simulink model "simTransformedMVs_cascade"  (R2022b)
settings: Solver=ode15s  StartTime=0.0  StopTime=tsim  RelTol=1e-3
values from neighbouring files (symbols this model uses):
  Kparu1 = [0 1]    [runTransformedMVs.m]    (also in runTransformedMVsIS.m)
  Kparu2 = [1 0]    [runTransformedMVs.m]    (also in runTransformedMVsIS.m)
  Ku1 = 1/ku1*1/(tauCu1)    (= -0.05)    [runTransformedMVs.m]    (also in runTransformedMVsIS.m = -2)
  Ku2 = 1/ku2*1/(tauCu2)    (= 0.5)    [runTransformedMVs.m]    (also in runTransformedMVsIS.m = 1)
  p = [V;A(i);B(i)]    [runTransformedMVs.m]    (also in runTransformedMVsIS.m; Main.m = [N, Fc0, rhoc, rhoh,U,A,cpc,cph]; Main_OL.m = [N, Fc0, rhoc, rhoh,U,A,cpc,cph]; runTestCalcBlk.m = [N, Fc0, rhoc, rhoh,U,A,cpc,cph])
  q10 = 5    [runTransformedMVs.m]    (also in runTransformedMVsIS.m)
  q1f = q10*1    (= 5)    [runTransformedMVs.m]    (also in runTransformedMVsIS.m)
  q1max = 10    [runTransformedMVs.m]    (also in runTransformedMVsIS.m)
  q20 = 5    [runTransformedMVs.m]    (also in runTransformedMVsIS.m)
  q2f = q20*1    (= 5)    [runTransformedMVs.m]    (also in runTransformedMVsIS.m = 5.5)
  q2max = 10    [runTransformedMVs.m]    (also in runTransformedMVsIS.m)
  T0 = 35    [runTransformedMVs.m]    (also in runTransformedMVsIS.m; H2P_Turbine_driven.m = param(9); runTD.m = 318; H2P_Boiler_driven.m = param(9))
  T10 = 20    [runTransformedMVs.m]    (also in runTransformedMVsIS.m)
  T1f = T10-5    (= 15)    [runTransformedMVs.m]    (also in runTransformedMVsIS.m = 25)
  T1fm = T10    (= 20)    [runTransformedMVs.m]    (also in runTransformedMVsIS.m = 25)
  T20 = 50    [runTransformedMVs.m]    (also in runTransformedMVsIS.m)
  T2f = T20    (= 50)    [runTransformedMVs.m]    (also in runTransformedMVsIS.m = 70)
  T2fm = T20    (= 50)    [runTransformedMVs.m]    (also in runTransformedMVsIS.m = 70)
  tauTs = 0.1    [runTransformedMVs.m]    (also in runTransformedMVsIS.m)
  td1 = 100    [runTransformedMVs.m]    (also in runTransformedMVsIS.m = 200)
  td2 = 150    [runTransformedMVs.m]    (also in runTransformedMVsIS.m = 300)
  tv1 = 50    [runTransformedMVs.m]    (also in runTransformedMVsIS.m = 100)
  tv2 = 50    [runTransformedMVs.m]    (also in runTransformedMVsIS.m = 100)
  v10 = q0    (= 10)    [runTransformedMVs.m]    (also in runTransformedMVsIS.m)
  v1f = q0    (= 10)    [runTransformedMVs.m]    (also in runTransformedMVsIS.m = 15)
  v20 = B(i)^(-1)*(f20-A(i)*T0)    [runTransformedMVs.m]    (also in runTransformedMVsIS.m; runTransfOL.m = v00)
  v2f = v20    [runTransformedMVs.m]    (also in runTransformedMVsIS.m)
undefined symbols (not defined in the file or in its folder): InputTransfD, TempMixDAE

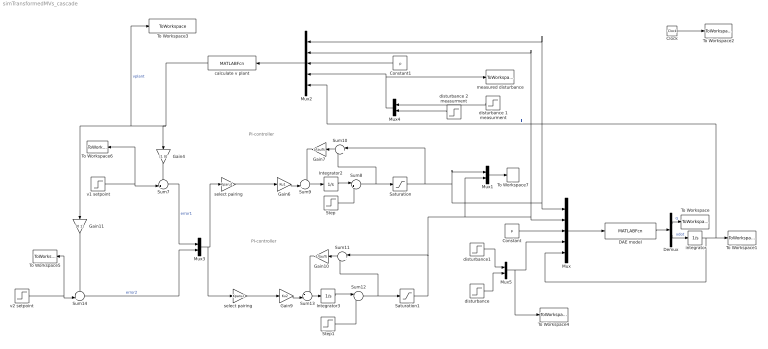
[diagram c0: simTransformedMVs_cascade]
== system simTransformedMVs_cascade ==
  note: PI-controller
  note: PI-controller
  " integrator" : Integrator  InitialCondition=T0
  Clock : Clock
  Constant : Constant  Value=p
  Constant1 : Constant  Value=p
  DAE model : MATLABFcn  MATLABFcn=TempMixDAE(u(1:2), u(3:5),u(6:7),u(8))  OutputDimensions=2
  Demux : Demux  Outputs=2
  Gain10 : Gain  Gain=1/tauTs  Multiplication=Matrix(K*u)
  Gain11 : Gain  Gain=[0 1]  Multiplication=Matrix(K*u)
  Gain4 : Gain  Gain=[1 0]  Multiplication=Matrix(K*u)
  Gain6 : Gain  Gain=Ku1  Multiplication=Matrix(K*u)
  Gain7 : Gain  Gain=1/tauTs  Multiplication=Matrix(K*u)
  Gain9 : Gain  Gain=Ku2  Multiplication=Matrix(K*u)
  Integrator2 : Integrator
  Integrator3 : Integrator
  Mux : Mux  Inputs=5
  Mux{1,3..5} (4 alike) : Mux  Inputs=2
  Mux2 : Mux  Inputs=5
  Saturation : Saturate  UpperLimit=q1max  LowerLimit=0
  Saturation1 : Saturate  UpperLimit=q2max  LowerLimit=0
  Step : Step  Time=tv1  Before=q10  After=q1f  SampleTime=0
  Step1 : Step  Time=tv2  Before=q20  After=q2f  SampleTime=0
  Sum10 : Sum  Inputs=|+-
  Sum11 : Sum  Inputs=|+-
  Sum12 : Sum  Inputs=|++
  Sum13 : Sum  Inputs=++|
  Sum14 : Sum  Inputs=-+|
  Sum7 : Sum  Inputs=-+|
  Sum8 : Sum  Inputs=|++
  Sum9 : Sum  Inputs=++|
  To Workspace : ToWorkspace  VariableName=q  SampleTime=-1
  To Workspace1 : ToWorkspace  VariableName=T  SampleTime=-1
  To Workspace2 : ToWorkspace  VariableName=time  SampleTime=-1
  To Workspace3 : ToWorkspace  VariableName=v  SampleTime=-1
  To Workspace4 : ToWorkspace  VariableName=d  SampleTime=-1
  To Workspace5 : ToWorkspace  VariableName=v2s  SampleTime=-1
  To Workspace6 : ToWorkspace  VariableName=v1s  SampleTime=-1
  To Workspace7 : ToWorkspace  VariableName=uplant  SampleTime=-1
  calculate v plant : MATLABFcn  MATLABFcn=InputTransfD(u(1:2),u(3:5),u(6:7),u(8))  OutputDimensions=2
  disturbance : Step  Time=td2  Before=T20  After=T2f  SampleTime=0
  disturbance 1 measurment : Step  Time=td1  Before=T10  After=T1fm  SampleTime=0
  disturbance 2 measurment : Step  Time=td2  Before=T20  After=T2fm  SampleTime=0
  disturbance1 : Step  Time=td1  Before=T10  After=T1f  SampleTime=0
  measured disturbance : ToWorkspace  VariableName=dm  SampleTime=-1
  select pairing : Gain  Gain=Kparu1  Multiplication=Matrix(K*u)
  "select pairing   " : Gain  Gain=Kparu2  Multiplication=Matrix(K*u)
  v1 setpoint : Step  Time=tv1  Before=v10  After=v1f  SampleTime=0
  v2 setpoint : Step  Time=tv2  Before=v20  After=v2f  SampleTime=0
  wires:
  DAE model/1 -> Demux/1
  Demux/1 -> To Workspace/1  "q"
  " integrator"/1 -> Mux2/5, To Workspace1/1, Mux/5  "T"
  Mux/1 -> DAE model/1
  Clock/1 -> To Workspace2/1
  v2 setpoint/1 -> To Workspace5/1, Sum14/2
  Demux/2 -> " integrator"/1  "xdot"
  calculate v plant/1 -> Gain11/1, To Workspace3/1, Gain4/1  "vplant"
  Saturation/1 -> Mux2/1, Mux/1, Mux1/1, Sum10/1
  Sum9/1 -> Integrator2/1
  Step/1 -> Sum8/2
  Gain7/1 -> Sum9/1
  Gain6/1 -> Sum9/2
  Gain4/1 -> Sum7/1
  Sum10/1 -> Gain7/1
  Sum8/1 -> Saturation/1, Sum10/2
  Sum12/1 -> Saturation1/1, Sum11/2
  Sum11/1 -> Gain10/1
  Saturation1/1 -> Mux2/2, Mux/2, Mux1/2, Sum11/1
  Gain9/1 -> Sum13/2
  Sum13/1 -> Integrator3/1
  Gain10/1 -> Sum13/1
  Gain11/1 -> Sum14/1
  Constant/1 -> Mux/3
  Mux1/1 -> To Workspace7/1
  Step1/1 -> Sum12/2
  v1 setpoint/1 -> To Workspace6/1, Sum7/2
  Sum7/1 -> Mux3/1  "error1"
  Sum14/1 -> Mux3/2  "error2"
  Mux2/1 -> calculate v plant/1
  Mux4/1 -> measured disturbance/1, Mux2/4
  Constant1/1 -> Mux2/3
  select pairing/1 -> Gain6/1
  Mux3/1 -> "select pairing   "/1, select pairing/1
  "select pairing   "/1 -> Gain9/1
  disturbance 2 measurment/1 -> Mux4/2
  disturbance 1 measurment/1 -> Mux4/1
  disturbance1/1 -> Mux5/1
  disturbance/1 -> Mux5/2
  Mux5/1 -> To Workspace4/1, Mux/4
  Integrator2/1 -> Sum8/1
  Integrator3/1 -> Sum12/1
